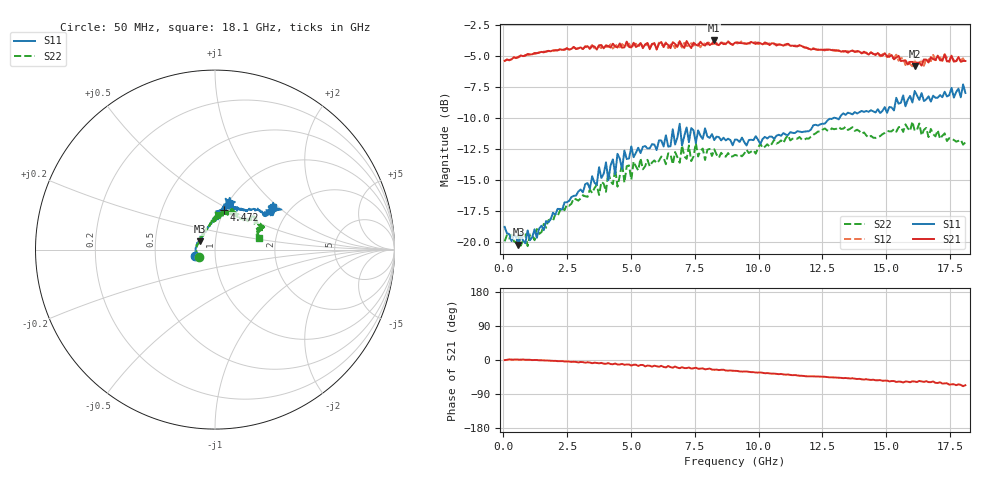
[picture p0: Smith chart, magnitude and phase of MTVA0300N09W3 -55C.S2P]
! Network Analyzer HP8720D.06.14 Serial No. US36140669
!  7 Jul 2005  12:40:01
! Frequency  S11  S21  S12  S22
# HZ  S  DB R 50
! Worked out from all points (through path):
!   201 points, 50 MHz to 18.1 GHz, reference 50 ohm
!   highest |S21| = -3.74 dB at 8.263 GHz (marker M1); lowest = -5.8 dB at 16.11 GHz (marker M2)
!   group delay of S21, straight-line fit = 11 ps
!   lowest |S11| = -20.2 dB at 591.5 MHz (marker M3), VSWR 1.22, Z = 42 + j4 ohm
!   |S11| at or under -10 dB: start of sweep to 12.94 GHz; 13.01 GHz to 13.17 GHz (160.2 MHz wide, 1.22 % of centre)
!   |S22| runs from -20.4 to -10.3 dB; largest |S21 - S12| = 0.041
!   S11 on the Smith chart (normalised r, x): 50 MHz: 0.80, -0.05; 4.472 GHz: 1.00, +0.47; 18.1 GHz: 1.63, +0.92
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5e7  -18.80 -163.1  -5.39 -0.3  -5.39 -0.2  -19.97 -155.0
5.915e8  -20.23 151.0  -5.10 0.9  -5.05 0.9  -19.52 154.9
9.525e8  -19.09 137.4  -4.82 0.6  -4.90 0.9  -20.36 139.8
3.1185e9  -16.00 92.8  -4.43 -5.6  -4.43 -6.2  -16.25 98.8
4.021e9  -13.59 85.2  -4.12 -10.1  -4.25 -8.5  -15.97 89.2
4.11125e9  -15.02 85.1  -4.20 -8.2  -4.25 -10.5  -14.35 87.7
4.382e9  -14.55 82.0  -4.23 -9.2  -4.18 -11.5  -14.10 87.5
4.47225e9  -12.90 76.7  -4.31 -11.8  -4.08 -9.8  -15.55 91.3
4.65275e9  -14.14 77.0  -4.33 -10.3  -4.03 -12.3  -13.66 89.2
4.743e9  -12.64 79.0  -4.29 -12.7  -4.23 -11.0  -15.23 85.5
5.104e9  -13.17 80.8  -3.92 -12.5  -4.06 -14.2  -13.52 79.7
6.09675e9  -11.81 73.6  -4.00 -17.9  -3.91 -17.5  -13.46 74.9
6.7285e9  -12.15 78.3  -4.02 -17.2  -4.35 -18.5  -12.75 67.5
6.909e9  -10.47 74.1  -3.79 -21.6  -3.95 -19.3  -13.62 66.9
6.99925e9  -12.22 74.3  -4.14 -19.1  -4.30 -21.8  -12.22 67.0
7.17975e9  -10.76 78.2  -3.78 -21.4  -4.16 -19.8  -13.31 61.9
8.26275e9  -11.79 71.9  -3.74 -25.7  -4.01 -26.7  -12.53 56.5
9.075e9  -11.74 67.8  -3.91 -28.6  -3.88 -28.8  -12.98 53.0
1.21435e10  -10.59 49.9  -4.42 -43.1  -4.36 -43.3  -11.36 42.2
1.512175e10  -9.11 33.1  -5.06 -56.5  -4.82 -56.1  -11.08 31.3
1.61145e10  -7.82 32.7  -5.84 -56.9  -5.33 -57.2  -11.04 27.8
1.81e10  -7.97 36.2  -5.40 -66.5  -5.64 -66.9  -11.98 15.2
